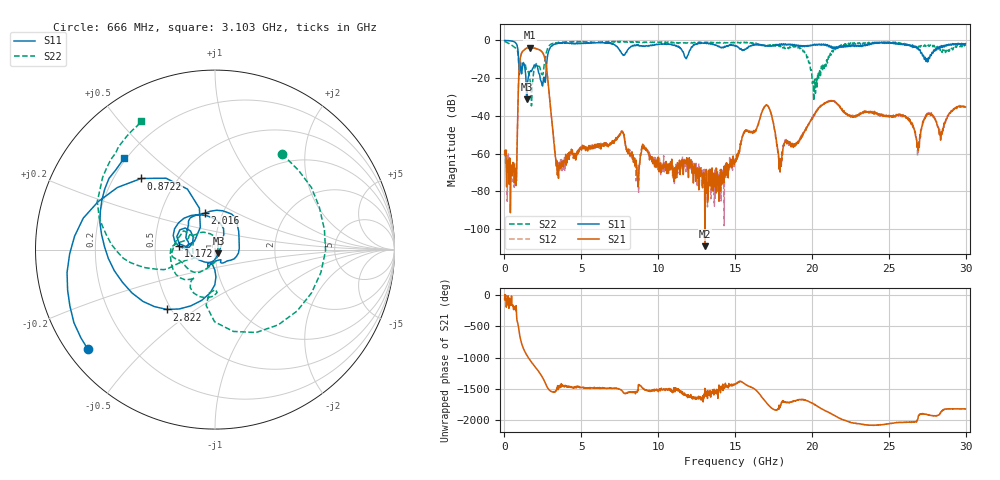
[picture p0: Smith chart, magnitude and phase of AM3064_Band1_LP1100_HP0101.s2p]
# Hz S DB R 50.0
!freq dBS11 angS11 dBS21 angS21 dBS12 angS12 dBS22 angS22
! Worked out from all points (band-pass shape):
!   1600 points, 10 MHz to 29.98 GHz, reference 50 ohm
!   highest |S21| = -3.77 dB at 1.678 GHz (marker M1); lowest = -109.0 dB at 13.04 GHz (marker M2)
!   |S21| within 3 dB of the highest: 1.112 GHz to 2.5 GHz (1.388 GHz wide, 76.8 % of centre)
!   lowest |S11| = -31.3 dB at 1.453 GHz (marker M3), VSWR 1.06, Z = 51.9 - j2.03 ohm
!   |S11| at or under -10 dB: 917 MHz to 2.775 GHz (1.858 GHz wide, 101 % of centre); 27.39404 GHz to 27.4591 GHz (65.05 MHz wide, 0.237 % of centre); 27.4884 GHz to 27.56287 GHz (74.48 MHz wide, 0.271 % of centre)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
!   |S22| runs from -34.7 to -0.5 dB; largest |S21 - S12| = 0.012
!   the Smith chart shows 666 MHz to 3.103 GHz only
!   S11 on the Smith chart (normalised r, x): 666 MHz: 0.06, -0.34; 872.2 MHz: 0.31, +0.37; 1.172 GHz: 0.66, +0.03; 2.016 GHz: 0.83, +0.35; 2.822 GHz: 0.48, -0.39; 3.103 GHz: 0.19, +0.40
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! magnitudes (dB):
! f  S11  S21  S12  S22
! 10 MHz  0.0  -60.2  -58.6  -0.5
! 666 MHz  -0.9  -70.3  -65.2  -3.7
! 872.2 MHz  -4.9  -36.3  -36.4  -6.6
! 1.172 GHz  -13.8  -5.9  -5.8  -13.2
! 1.453 GHz  -31.3  -4.1  -4.0  -15.9
! 1.678 GHz  -16.4  -3.8  -3.8  -22.1
! 2.016 GHz  -13.5  -4.2  -4.2  -13.6
! 2.822 GHz  -7.4  -20.9  -20.8  -3.9
! 3.103 GHz  -2.9  -44.3  -44.4  -1.7
! 3.496 GHz  -1.6  -68.9  -67.4  -1.2
! 5.015 GHz  -1.6  -58.2  -57.1  -0.6
! 7.62 GHz  -6.9  -48.5  -48.5  -0.7
! 8.613 GHz  -2.6  -70.4  -68.0  -1.0
! 10 GHz  -2.1  -61.8  -64.8  -1.0
! 13.04 GHz  -1.5  -109.0  -68.9  -1.2
! 15 GHz  -3.0  -64.5  -64.8  -1.4
! 16.99 GHz  -3.0  -34.6  -34.5  -2.7
! 17.93 GHz  -2.0  -69.7  -63.9  -2.8
! 19.99 GHz  -2.8  -41.5  -41.8  -18.1
! 25 GHz  -1.0  -40.4  -40.1  -1.2
! 26.89 GHz  -4.0  -56.9  -54.4  -3.3
! 29.98 GHz  -1.7  -35.3  -35.2  -2.9
